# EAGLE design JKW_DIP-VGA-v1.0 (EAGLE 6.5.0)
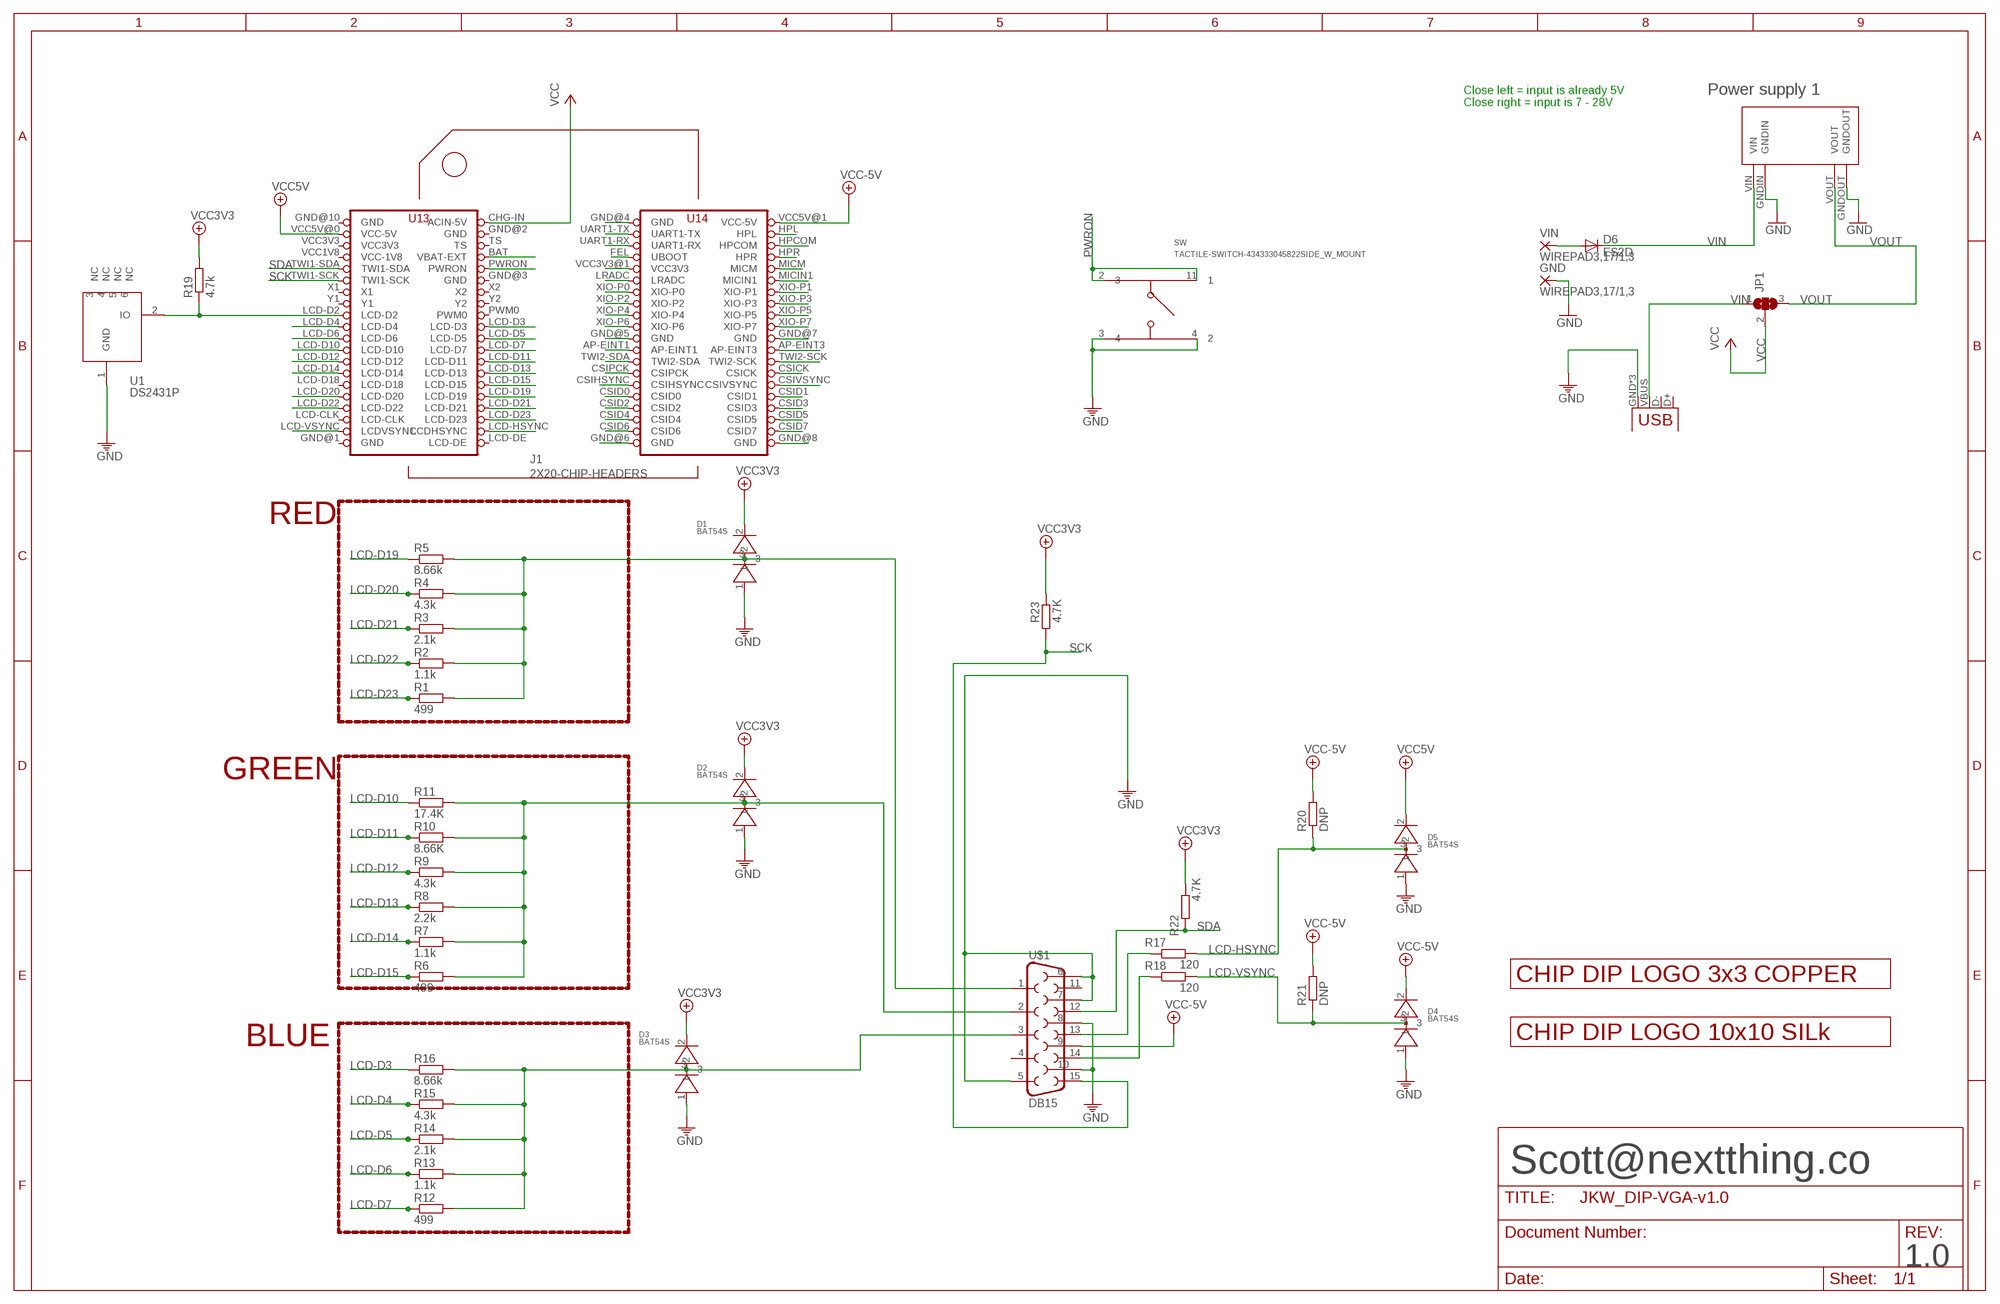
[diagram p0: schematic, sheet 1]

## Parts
D1  BAT54S  [SOT23-BEC]
D2  BAT54S  [SOT23-BEC]
D3  BAT54S  [SOT23-BEC]
D4  BAT54S  [SOT23-BEC]
D5  BAT54S  [SOT23-BEC]
D6  ES2D  [SMB]
GND  WIREPAD3,17/1,3  [3,17/1,3]
J1  2X20-CHIP-HEADERS  [2X20CHIP_SM]
JP1  SJ2W  [SJ_2]
R1  499  R-EU_R0805  [R0805]
R2  1.1k  R-EU_R0805  [R0805]
R3  2.1k  R-EU_R0805  [R0805]
R4  4.3k  R-EU_R0805  [R0805]
R5  8.66k  R-EU_R0805  [R0805]
R6  499  R-EU_R0805  [R0805]
R7  1.1k  R-EU_R0805  [R0805]
R8  2.2k  R-EU_R0805  [R0805]
R9  4.3k  R-EU_R0805  [R0805]
R10  8.66K  R-EU_R0805  [R0805]
R11  17.4K  R-EU_R0805  [R0805]
R12  499  R-EU_R0805  [R0805]
R13  1.1k  R-EU_R0805  [R0805]
R14  2.1k  R-EU_R0805  [R0805]
R15  4.3k  R-EU_R0805  [R0805]
R16  8.66k  R-EU_R0805  [R0805]
R17  120  R-EU_R0805  [R0805]
R18  120  R-EU_R0805  [R0805]
R19  4.7k  R-EU_R0805  [R0805]
R20  DNP  R-EU_R0805  [R0805]
R21  DNP  R-EU_R0805  [R0805]
R22  4.7K  R-EU_R0805  [R0805]
R23  4.7K  R-EU_R0805  [R0805]
SW  TACTILE-SWITCH-434333045822SIDE_W_MOUNT  [TACTILE-SWITCH-K2-1114UA-AW]
U1  DS2431P  [TSOC6]
U$1  DB15  [DB15]
U$5  LOGO_3X3_COPPER  [LOGO_3X3_COPPER]
U$6  LOGO_10X10_SILK  [LOGO_10X10_SILK]
U$9  MP1584EN  [MP1584EN]
USB  USBUSB-MICROB-SMT-DIP  [USB-MICROB-SMT-DIP]
VIN  WIREPAD3,17/1,3  [3,17/1,3]

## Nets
1: J1.CSIVSYNC
AP-EINT1: J1.AP-EINT1
AP-EINT3: J1.AP-EINT3
BAT: J1.BAT(VBAT-EXT)
CSICK: J1.CSICK
CSID0: J1.CSID0
CSID1: J1.CSID1
CSID2: J1.CSID2
CSID3: J1.CSID3
CSID4: J1.CSID4
CSID5: J1.CSID5
CSID6: J1.CSID6
CSID7: J1.CSID7
CSIHSYNC: J1.CSIHSYNC
CSPICK: J1.CSIPCK
FEL: J1.FEL(UBOOT)
GND: D1.1 D2.1 D3.1 D4.1 D5.1 GND.1(P) J1.GND@4(GND) J1.GND@5(GND) J1.GND@6(GND) J1.GND@7(GND) J1.GND@8(GND) SW.3 SW.4 U1.1(GND) U$1.5 U$1.6 U$1.7 U$1.8 U$1.10 U$9.GNDIN U$9.GNDOUT USB.GND USB.MT1(GND) USB.MT2(GND)
HPCOM: J1.HPCOM
HPL: J1.HPL
HPR: J1.HPR
LCD-D3: J1.LCD-D3 R16.1
LCD-D4: J1.LCD-D4 R15.1
LCD-D5: J1.LCD-D5 R14.1
LCD-D6: J1.LCD-D6 R13.1
LCD-D7: J1.LCD-D7 R12.1
LCD-D10: J1.LCD-D10 R11.1
LCD-D11: J1.LCD-D11 R10.1
LCD-D12: J1.LCD-D12 R9.1
LCD-D13: J1.LCD-D13 R8.1
LCD-D14: J1.LCD-D14 R7.1
LCD-D15: J1.LCD-D15 R6.1
LCD-D19: J1.LCD-D19 R5.1
LCD-D20: J1.LCD-D20 R4.1
LCD-D21: J1.LCD-D21 R3.1
LCD-D22: J1.LCD-D22 R2.1
LCD-D23: J1.LCD-D23 R1.1
LCD-HSYNC: D5.3 J1.LCD-HSYNC(LCDHSYNC) R17.2 R20.1
LCD-VSYNC: D4.3 J1.LCD-VSYNC(LCDVSYNC) R18.2 R21.1
LRADC: J1.LRADC
MICIN1: J1.MICIN1
MICM: J1.MICM
N$1: R17.1 U$1.13
N$2: R18.1 U$1.14
N$3: JP1.1 USB.VBUS
N$5: J1.LCD-D2 R19.1 U1.2(IO)
N$12: D2.3 R6.2 R7.2 R8.2 R9.2 R10.2 R11.2 U$1.2
N$13: D1.3 R1.2 R2.2 R3.2 R4.2 R5.2 U$1.1
N$19: D3.3 R12.2 R13.2 R14.2 R15.2 R16.2 U$1.3
N$65: D6.A VIN.1(P)
PWRON: J1.PWRON SW.2 SW.11
SCK: J1.TWI1-SCK R23.1 U$1.15
SDA: J1.TWI1-SDA R22.1 U$1.12
TWI2-SCK: J1.TWI2-SCK
TWI2-SDA: J1.TWI2-SDA
UART1-RX: J1.UART1-RX
UART1-TX: J1.UART1-TX
VCC: J1.CHG-IN(ACIN-5V) JP1.2
VCC3V3: D1.2 D2.2 D3.2 J1.VCC3V3@1(VCC3V3) R19.2 R22.2 R23.2
VCC5V: D4.2 D5.2 J1.VCC5V@0(VCC-5V) J1.VCC5V@1(VCC-5V) R20.2 R21.2 U$1.9 ; supply symbol labelled VCC-5V
VIN: D6.C U$9.VIN
VOUT: JP1.3 U$9.VOUT
XIO-P0: J1.XIO-P0
XIO-P1: J1.XIO-P1
XIO-P2: J1.XIO-P2
XIO-P3: J1.XIO-P3
XIO-P4: J1.XIO-P4
XIO-P5: J1.XIO-P5
XIO-P6: J1.XIO-P6
XIO-P7: J1.XIO-P7
Unconnected: J1.LCD-CLK J1.LCD-D18 J1.LCD-DE J1.PWM0 J1.TS J1.X1 J1.X2 J1.Y1 J1.Y2 U1.3(NC) U1.4(NC) U1.5(NC) U1.6(NC) U$1.4 U$1.11 USB.D+ USB.D-

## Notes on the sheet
- Power supply 1
- Close left = input is already 5V
  Close right = input is 7 - 28V
- RED
- GREEN
- BLUE
- Scott@nextthing.co
- 1.0

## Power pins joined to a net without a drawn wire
GND: J1.GND@1(GND) J1.GND@2(GND) J1.GND@3(GND) J1.GND@10(GND)
VCC3V3: J1.VCC3V3
VCC-1V8: J1.VCC1V8(VCC-1V8)

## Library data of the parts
D1-D5 = VGA-DIP:BAT54S
D6 = diode:ES2D: DIODE
GND VIN = wirepad:WIREPAD: Wire PAD connect wire on PCB
J1 = VGA-DIP:2X20-CHIP-HEADERS: Through hole layout with chip reference
JP1 = jumper:SJ2W: SMD solder JUMPER
R1-R23 = rcl:R-EU_: RESISTOR, European symbol
SW = cheeper:TACTILE-SWITCH-434333045822
U1 = VGA-DIP:DS2431: 1024-Bit EEPROM This chip provides a 4x256 Bit EEPROM, which can be programmed@5V. Write protection and OTP emulation are available, too. Author: Jan Kandziora <jjj@gmx.de>; DESCRIPTION: IC, 1024-Bit, 1-Wire EEPROM, TSOC6; FOOTPRINT: TSOC6; LINK: http://www.digikey.com/product-detail/en/DS2431P%2BT%26R/DS2431P%2BT%26RCT-ND/3647900; MFG: DIGIKEY; MFG_PN: DS2431P+T&RCT-ND; PART_TYPE: IC; PRICE: 0.98; VENDOR: MAXIM; VENDOR_PART_NUMBER: DS2431P+T&R
U$1 = SparkFun-Connectors:DB15: DB15 / VGA right angle through-hole female connector.
U$5 = logo:LOGO_3X3_COPPER
U$6 = logo:LOGO_10X10_SILK
U$9 = power_supply:MP1584EN
USB = Spark:USB

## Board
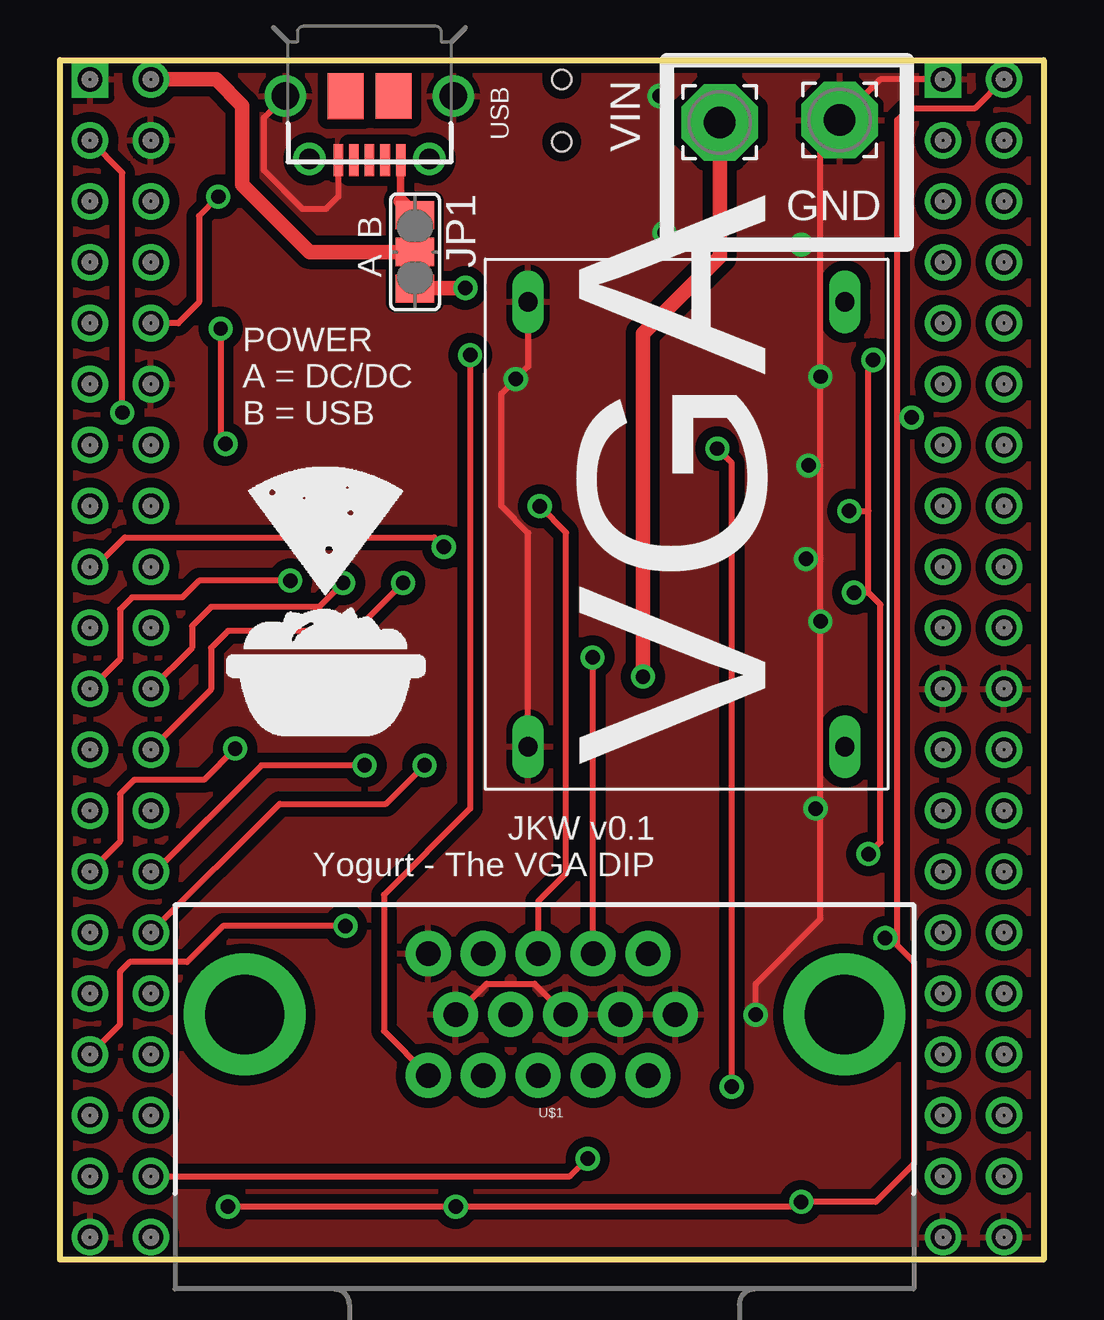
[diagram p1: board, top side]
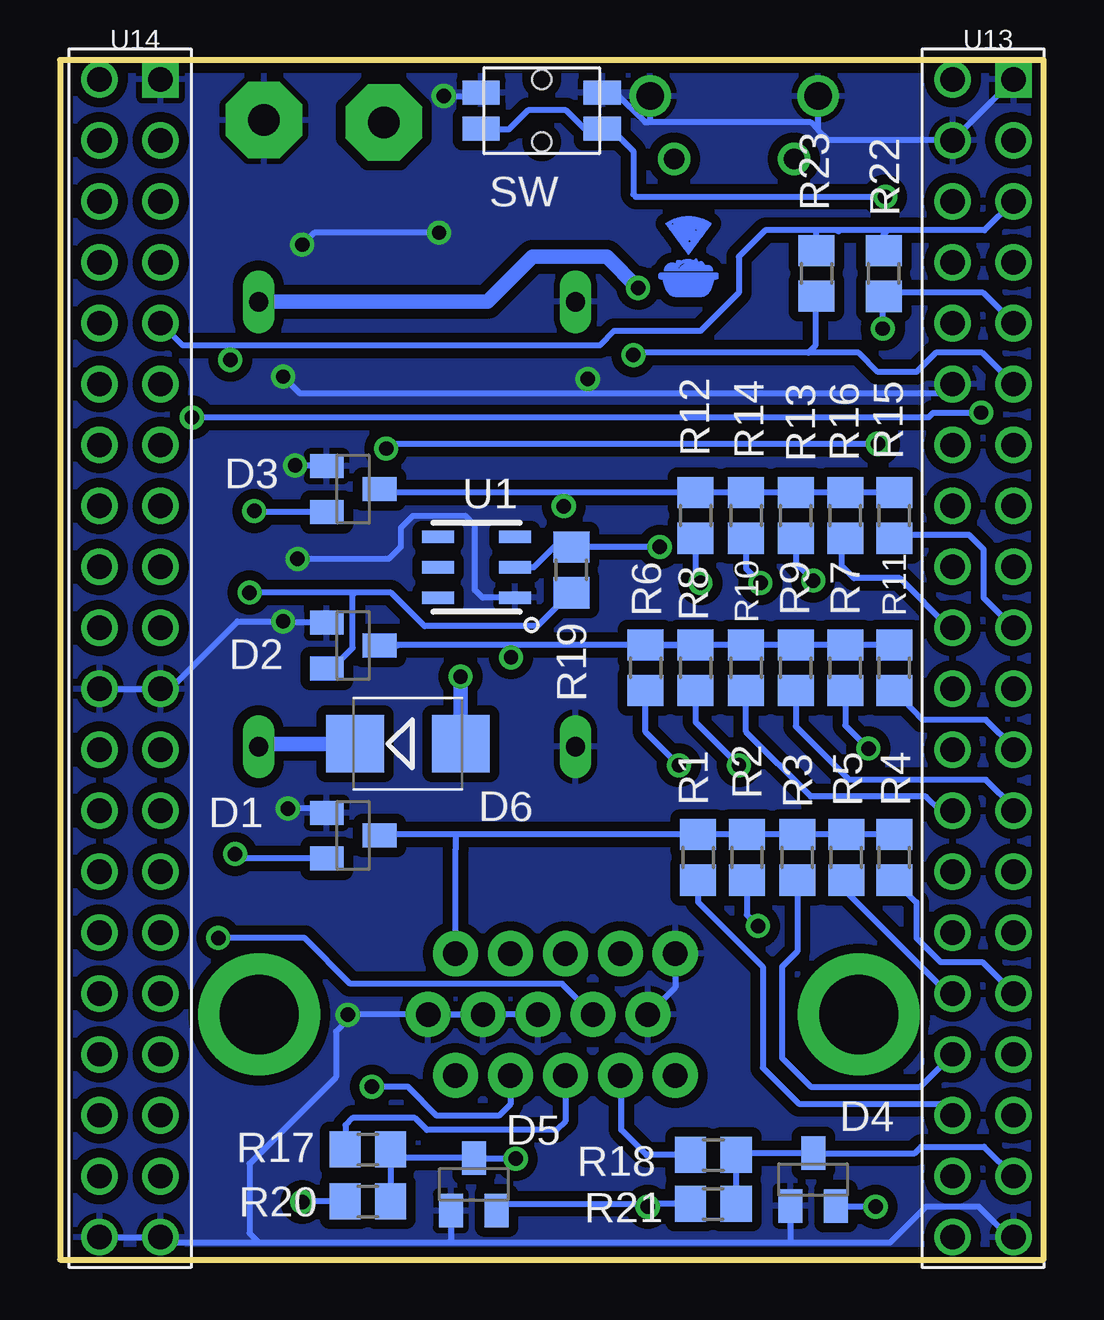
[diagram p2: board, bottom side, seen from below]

Size 41 x 50 mm. Coordinates in mm from the lower left corner, seen from the top.
Outline: 41,0 0,0 0,50 41,50 41,0
Copper layers (1*2*15*16): Top 0.035mm / dielectric 0.2mm / Route2 0.035mm / dielectric 0.2mm / Route15 0.035mm / dielectric 0.2mm / Bottom 0.035mm
Design rules "Hampoo *": minimum track width 3mil, minimum drill 8mil, track to track 3mil, track to pad 3mil, pad to pad 3mil, via to via 3mil, smd to smd 3mil, copper to edge 10mil, drill to drill 8mil, minimum pad ring 10mil, minimum via ring 8mil, stop-mask expansion 4mil, vias tented up to drill 39mil, thermal gap 10mil

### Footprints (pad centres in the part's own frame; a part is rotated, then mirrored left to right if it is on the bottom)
SOT23-BEC = smd 1 x 1.4: 1 -0.95,-1.1; 2 0.95,-1.1; 3 0,1.1
SMB = smd 2.4 x 2.4: A 2.2,0; C -2.2,0
3,17/1,3 = drill 1.321 pad 3.175 octagon: 1 0,0
2X20CHIP_SM = drill 1.016: AP-EINT1 36.81,21.65; AP-EINT3 39.35,21.65; BAT 3.79,41.97; CHG-IN 3.79,49.59; CSICK 39.35,16.57; CSID0 36.81,11.49; CSID1 39.35,11.49; CSID2 36.81,8.95; CSID3 39.35,8.95; CSID4 36.81,6.41; CSID5 39.35,6.41; CSID6 36.81,3.87; CSID7 39.35,3.87; CSIHSYNC 36.81,14.03; CSIPCK 36.81,16.57; CSIVSYNC 39.35,14.03; FEL 36.81,41.97; GND@1 3.79,36.89; GND@2 1.25,1.33; GND@4 39.35,24.19; GND@5 39.35,1.33; GND@6 36.81,1.33; GND@7 36.81,24.19; GND@10 3.79,47.05; HPCOM 39.35,44.51; HPL 39.35,47.05; HPR 39.35,41.97; LCD-CLK 1.25,6.41; LCD-D2 1.25,29.27; LCD-D3 3.79,26.73; LCD-D4 1.25,26.73; LCD-D5 3.79,24.19; LCD-D6 1.25,24.19; LCD-D7 3.79,21.65; LCD-D10 1.25,21.65; LCD-D11 3.79,19.11; LCD-D12 1.25,19.11; LCD-D13 3.79,16.57; LCD-D14 1.25,16.57; LCD-D15 3.79,14.03; LCD-D18 1.25,14.03; LCD-D19 3.79,11.49; LCD-D20 1.25,11.49; LCD-D21 3.79,8.95; LCD-D22 1.25,8.95; LCD-D23 3.79,6.41; LCD-DE 3.79,1.33; LCD-HSYNC 3.79,3.87; LCD-VSYNC 1.25,3.87; LRADC 36.81,36.89; MICIN1 39.35,36.89; MICM 39.35,39.43; PWM0 3.79,29.27; PWRON 3.79,39.43; TS 3.79,44.51; TWI1-SCK 1.25,36.89; TWI1-SDA 1.25,39.43; TWI2-SCK 39.35,19.11; TWI2-SDA 36.81,19.11; UART1-RX 36.81,44.51; UART1-TX 36.81,47.05; VCC1V8 1.25,41.97; VCC3V3 1.25,44.51; VCC3V3@1 36.81,39.43; VCC5V@0 1.25,47.05; VCC5V@1 39.35,49.59; X1 1.25,34.35; X2 3.79,34.35; XIO-P0 36.81,34.35; XIO-P1 39.35,34.35; XIO-P2 36.81,31.81; XIO-P3 39.35,31.81; XIO-P4 36.81,29.27; XIO-P5 39.35,29.27; XIO-P6 36.81,26.73; XIO-P7 39.35,26.73; Y1 1.25,31.81; Y2 3.79,31.81 | drill 1.016 square: GND@3 1.25,49.59; GND@8 36.81,49.59
SJ_2 = smd 1.168 x 1.6: 1 -1.524,0; 2 0,0; 3 1.524,0
R0805 = smd 1.3 x 1.5: 1 -0.95,0; 2 0.95,0
TACTILE-SWITCH-K2-1114UA-AW = smd 1.55 x 1: 2 -2.525,0.75; 3 -2.525,-0.75; 4 2.525,-0.75; 11 2.525,0.75 | hole 0.8: 0,1.3; 0,-1.3
TSOC6 = smd 0.53 x 1.33: 1 -1.27,-1.6; 2 0,-1.6; 3 1.27,-1.6; 4 1.27,1.6; 5 0,1.6; 6 -1.27,1.6
DB15 = drill 1.016 pad 1.88: 1 -4.32,-7.62; 2 -2.03,-7.62; 3 0.26,-7.62; 4 2.55,-7.62; 5 4.84,-7.62; 6 -5.46,-5.08; 7 -3.17,-5.08; 8 -0.88,-5.08; 9 1.41,-5.08; 10 3.7,-5.08; 11 -4.32,-2.54; 12 -2.03,-2.54; 13 0.26,-2.54; 14 2.55,-2.54; 15 4.84,-2.54 | drill 3.302 pad 5.08: G1 -12.5,-5.08; G2 12.5,-5.08
MP1584EN = drill 0.8 long: GNDIN 1.778,14.986; GNDOUT 20.32,14.986; VIN 1.778,1.778; VOUT 20.32,1.778
USB-MICROB-SMT-DIP = smd 0.4 x 1.35: D+ 0,2.675; D- -0.65,2.675; GND 1.3,2.675; ID 0.65,2.675; VBUS -1.3,2.675 | drill 1.15 pad 1.7: MT1 -3.5,0; MT2 3.5,0 | drill 0.85 pad 1.25: MT3 -2.5,2.625; MT4 2.5,2.625 | smd 1.5 x 1.9: P$1 -1,0; P$2 1,0.01

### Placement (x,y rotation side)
D1  28.78,17.68 270 bottom
D2  28.78,25.6 270 bottom
D3  28.78,32.12 270 bottom
D4  9.6,3.33 0 bottom
D5  23.75,3.13 0 bottom
D6  26.5,21.5 0 bottom
GND  32.5,47.5 0 top
J1  0,-0.4 0 top
JP1  14.8,42 270 top
R1  14.4,16.76 90 bottom
R2  12.37,16.76 90 bottom
R3  10.27,16.76 90 bottom
R4  6.22,16.76 90 bottom
R5  8.22,16.76 90 bottom
R6  16.59,24.66 90 bottom
R7  8.27,24.66 90 bottom
R8  14.51,24.66 90 bottom
R9  10.32,24.66 90 bottom
R10  12.4,24.66 90 bottom
R11  6.22,24.66 90 bottom
R12  14.51,31.01 90 bottom
R13  10.32,31.01 90 bottom
R14  12.4,31.01 90 bottom
R15  6.22,31.01 90 bottom
R16  8.27,31.01 90 bottom
R17  28.16,4.59 0 bottom
R18  13.76,4.35 0 bottom
R19  19.69,28.75 270 bottom
R20  28.17,2.42 180 bottom
R21  13.77,2.32 180 bottom
R22  6.67,41.1 90 bottom
R23  9.47,41.1 90 bottom
SW  20.92,47.89 180 bottom
U1  23.63,28.86 90 bottom
U$1  20.19,5.13 180 top
U$5  14.8,41.8 0 bottom
U$6  6.9,21.8 0 top
U$9  34.5,19.6 90 top
USB  12.9,48.5 180 top
VIN  27.5,47.4 0 top

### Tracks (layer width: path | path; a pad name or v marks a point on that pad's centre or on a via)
GND  (via drill 0.6)
  Top 0.254: U$1.10 17.78,11.5 19.78,11.5 U$1.8 | 31.7,29.2 v31.7,26.6 31.7,19 | 31.7,29.2 31.7,33.1 | 31.7,33.1 v31.7,36.8 31.7,42.3 | v31.2,33.1 31.7,33.1 | v31.5,18.8 31.7,19 | v29,10.2 29,11.5 31.7,14.2 31.7,19 | v31.1,29.2 31.7,29.2 | USB.GND 11.6,44.3 11.1,43.8 10.1,43.8 8.5,45.4 8.5,47.6 USB.MT2 | v30.9,42.3 31.7,42.3 | U$9.GNDIN 19.51,30.29 18.4,31.4 18.4,36.1 v19,36.7 19.51,37.21 U$9.GNDOUT | 31.7,42.3 31.7,46.7 GND.1 34.19,49.19 J1.GND@8 | v25.2,42.8 25.2,48.3 v25,48.5
  Bottom 0.254: U$1.8 U$1.7 U$1.6 28.79,10.21 28.8,10.2 | J1.GND@5 J1.GND@6 36.58,0.7 32.7,0.7 | J1.GND@2 1.43,0.93 2.7,2.2 4.9,2.2 6.4,0.7 10.6,0.7 | 10.6,0.7 24.8,0.7 | 24.8,0.7 32.7,0.7 | D4.1 10.55,0.75 10.6,0.7 | D5.1 24.7,0.8 24.8,0.7 | 28.8,10.2 29.5,9.5 29.5,7.6 33.1,4 33.1,1.1 32.7,0.7 | U$1.5 15.35,11.35 U$1.10 | D2.1 31.64,26.55 v31.7,26.6 33.6,26.6 36.41,23.79 J1.GND@7 J1.GND@4 | D3.1 29.91,33.1 v31.2,33.1 | D1.1 30.05,18.8 v31.5,18.8 | 28.8,10.2 v29,10.2 | J1.GND@3 J1.GND@10 8.95,46.65 9.4,47.1 | J1.GND@1 4.18,36.1 19,36.1 | 19,36.1 31,36.1 v31.7,36.8 | U1.1 23.39,27.59 23.7,27.9 23.7,30.6 24.1,31 26.3,31 26.8,30.5 26.8,29.7 27.3,29.2 v31.1,29.2 | 9.4,47.1 9.7,47.4 16.5,47.4 | USB.MT2 9.4,47.1 | USB.MT1 16.4,47.5 16.5,47.4 | 16.5,47.4 16.6,47.4 17.84,48.64 SW.3 | v19,36.7 19,36.1 | v25,48.5 23.58,48.5 SW.4 | v25.2,42.8 30.4,42.8 v30.9,42.3
  pour Top (isolate 0.406): 0,0 41,0 41,50 0,50
  pour Bottom (isolate 0.406): 0,0 41,0 41,50 0,50
LCD-D3
  Bottom 0.254: J1.LCD-D3 3.93,26.33 6,28.4 7.9,28.4 8.4,28.9 8.4,30.04 R16.1
LCD-D4
  Bottom 0.254: J1.LCD-D4 2.5,27.58 2.5,29.6 3.1,30.2 6.25,30.2 R15.1
LCD-D5  (via drill 0.6)
  Top 0.254: v11.8,28.2 10.8,27.2 6.3,27.2 5.5,26.4 5.5,25.5 J1.LCD-D5
  Bottom 0.254: R14.1 12.4,28.8 v11.8,28.2
LCD-D6  (via drill 0.6)
  Top 0.254: v9.6,28.3 5.8,28.3 5.1,27.6 3,27.6 2.5,27.1 2.5,25.04 J1.LCD-D6
  Bottom 0.254: R13.1 10.32,29.03 v9.6,28.3
LCD-D7  (via drill 0.6)
  Top 0.254: v14.3,28.2 12.3,26.2 7,26.2 6.3,25.5 6.3,23.76 J1.LCD-D7
  Bottom 0.254: R12.1 14.51,28.41 v14.3,28.2
LCD-D10
  Bottom 0.254: J1.LCD-D10 1.25,21.35 2.4,22.5 5.05,22.5 R11.1
LCD-D11
  Bottom 0.254: J1.LCD-D11 4.31,18.71 4.9,19.3 9.7,19.3 12.4,22 R10.1
LCD-D12
  Bottom 0.254: J1.LCD-D12 1.25,18.85 2.4,20 8.1,20 10.1,22 10.2,22.1 10.32,22.23 R9.1
LCD-D13  (via drill 0.6)
  Top 0.254: v12.7,20.6 8.4,20.6 3.97,16.17 J1.LCD-D13
  Bottom 0.254: R8.1 14.51,22.41 v12.7,20.6
LCD-D14  (via drill 0.6)
  Top 0.254: v7.3,21.3 6,20 3.1,20 2.5,19.4 2.5,17.42 J1.LCD-D14
  Bottom 0.254: R7.1 8.27,22.27 v7.3,21.3
LCD-D15  (via drill 0.6)
  Top 0.254: J1.LCD-D15 9.16,19 13.6,19 v15.2,20.6
  Bottom 0.254: v15.2,20.6 16.59,21.99 R6.1
LCD-D19
  Bottom 0.254: J1.LCD-D19 3.99,11.09 8.22,15.32 R5.1
LCD-D20
  Bottom 0.254: R4.1 5.3,14.89 5.3,13.4 4.3,12.4 2.56,12.4 J1.LCD-D20
LCD-D21
  Bottom 0.254: R3.1 10.27,12.83 10.9,12.2 10.9,8.4 9.7,7.2 5.14,7.2 J1.LCD-D21
LCD-D22  (via drill 0.6)
  Top 0.254: v11.9,13.9 6.8,13.9 5.3,12.4 2.9,12.4 2.65,12.15 2.6,12.1 2.5,12 2.5,9.8 J1.LCD-D22
  Bottom 0.254: R2.1 12.37,14.37 v11.9,13.9
LCD-D23
  Bottom 0.254: R1.1 14.4,14.9 11.7,12.2 11.7,8 10.2,6.5 4.28,6.5 J1.LCD-D23
LCD-HSYNC  (via drill 0.6)
  Top 0.254: J1.LCD-HSYNC 21.27,3.47 v22,4.2
  Bottom 0.254: R20.1 R17.2 26.86,4.23 D5.3 23.71,4.2 v22,4.2
LCD-VSYNC
  Bottom 0.254: J1.LCD-VSYNC 2.48,4.7 5.1,4.7 5.37,4.43 D4.3 12.73,4.43 R18.2 R21.1
N$1
  Bottom 0.254: U$1.13 19.93,5.77 20.3,5.4 25.7,5.4 26.2,5.9 28.8,5.9 29.1,5.6 29.1,4.6 R17.1
N$2
  Bottom 0.254: R18.1 16.55,4.35 17.6,5.4 17.6,7.63 U$1.14
N$3
  Top 0.305: USB.VBUS 14.2,44.12
  Top 0.61: 14.2,44.12 JP1.1
N$5  (via drill 0.6)
  Top 0.254: J1.LCD-D2 1.47,28.87 2.7,30.1 15.6,30.1 v16,29.7
  Bottom 0.254: U1.2 21.25,28.86 20.4,29.7 R19.1 v16,29.7
N$12  (via drill 0.6)
  Top 0.254: v22.2,25.1 22.22,25.08 U$1.2
  Bottom 0.254: R11.2 R7.2 R9.2 R10.2 R6.2 R8.2 22.2,25.61 | 22.2,25.61 26.9,25.61 | 26.9,25.61 26.99,25.61 27,25.6 | D2.3 26.92,25.6 26.9,25.61 | v22.2,25.1 22.2,25.61
N$13
  Bottom 0.254: R4.2 R5.2 R3.2 R2.2 R1.2 24.5,17.71 | 24.5,17.71 27.59,17.71 27.62,17.68 D1.3 | 24.5,17.71 24.5,17.1 24.51,17.09 U$1.1
N$19  (via drill 0.6)
  Top 0.254: 19.93,31.33 v20,31.4 21.1,30.3 21.1,16.1 19.93,14.93 U$1.3
  Bottom 0.254: R16.2 R13.2 R14.2 R12.2 20,31.96 | 20,31.96 27.53,31.96 D3.3 | R15.2 R16.2 | R16.2 8.27,31.94 8.3,31.9 | v20,31.4 20,31.96
N$65  (via drill 0.6)
  Top 0.61: v24.3,24.3 24.3,38.6 27.5,41.8 VIN.1
  Bottom 0.61: D6.A v24.3,24.3
PWRON  (via drill 0.6)
  Top 0.254: v6.6,44.3 5.8,43.5 5.8,39.9 4.93,39.03 J1.PWRON
  Bottom 0.254: v6.6,44.3 17,44.3 17.1,44.4 17.1,46.2 18.04,47.14 SW.2 19.14,47.14 19.9,47.9 21.5,47.9 22.3,47.1 23.41,47.1 SW.11
SCK  (via drill 0.6)
  Top 0.254: v17.1,37.7 17.1,18.8 13.5,15.2 13.5,9.52 U$1.15
  Bottom 0.254: J1.TWI1-SCK 2.56,37.8 4.5,37.8 5.3,37 6.9,37 7.7,37.8 9.8,37.8 | 9.5,40.12 R23.1 9.52,40.2 9.52,38.09 9.8,37.8 | 9.8,37.8 17,37.8 v17.1,37.7
SDA  (via drill 0.6)
  Top 0.254: v28,7.2 28,33.2 v27.4,33.8 | v6.7,38.8 6.7,34.2 arc90 v6.9,34
  Bottom 0.254: J1.TWI1-SDA 2.52,40.3 6.61,40.3 R22.1 6.7,40.11 v6.7,38.8 | U$1.12 22.22,6.48 22.7,6 25.3,6 26.5,7.2 v28,7.2 | v6.9,34 27.2,34 arc-90 v27.4,33.8
VCC
  Top 0.61: J1.CHG-IN 6.51,49.19 7.6,48.1 7.6,44.8 10.4,42 JP1.2
VCC3V3  (via drill 0.6)
  Top 0.254: 33.7,27.8 33.7,31.2 | v32.9,31.2 33.7,31.2 | v33.1,27.8 33.7,27.8 | 33.7,27.8 34.2,27.3 34.2,17.4 v33.7,16.9 | 33.7,31.2 33.7,37.3 v33.9,37.5
  Bottom 0.254: J1.VCC3V3 2.46,42.9 6.5,42.9 | 6.5,42.9 8.6,42.9 | 8.6,42.9 9.5,42.9 | 8.55,42.85 8.6,42.9 | R22.2 6.67,42.73 6.5,42.9 | R23.2 9.47,42.87 9.5,42.9 | D1.2 33.52,16.73 v33.7,16.9 | 36.74,39.1 J1.VCC3V3@1 35.88,38.1 33.9,38.1 | D3.2 32.87,31.17 v32.9,31.2 | 9.5,42.9 11.6,42.9 12.7,41.8 12.7,40.3 14.3,38.7 17.9,38.7 18.5,38.1 33.9,38.1 | R19.2 19.7,27.8 21.1,26.4 25.8,26.4 27.2,27.8 28.7,27.8 | 28.7,27.8 v33.1,27.8 | D2.2 29.66,24.65 28.8,25.5 28.8,27.7 28.7,27.8 | v33.9,37.5 33.9,38.1
VCC5V  (via drill 0.6)
  Top 0.254: 34.9,13.4 34.9,13.1 35.6,12.4 35.6,4 34,2.4 v30.9,2.4 30.7,2.2 v16.5,2.2 v7,2.2 | 34.9,13.4 34.9,35.1 | 34.9,35.1 34.9,47.5 35.4,48 38.16,48 J1.VCC5V@1 | v34.4,13.4 34.9,13.4 | v35.5,35.1 34.9,35.1 | v2.6,35.3 2.6,45.3 J1.VCC5V@0
  Bottom 0.254: U$1.9 20.07,11.5 28.9,11.5 30.8,13.4 v34.4,13.4 | R20.2 30.88,2.42 v30.9,2.4 | v35.5,35.1 4.8,35.1 4.6,35.3 v2.6,35.3 | D5.2 22.87,2.03 | 22.87,2.03 22.9,2 | v7,2.2 8.62,2.2 D4.2 | R21.2 16.38,2.32 | 16.38,2.32 v16.5,2.2 | 22.87,2.03 22.58,2.32 16.38,2.32
VIN
  Bottom 0.61: D6.C 32.6,21.5 arc-90 U$9.VIN
VOUT  (via drill 0.6)
  Top 0.61: v16.9,40.5 14.82,40.5 JP1.3
  Bottom 0.61: U$9.VOUT 23.18,39.92 21.3,41.8 18.2,41.8 v16.9,40.5

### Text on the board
tNames: B | A | POWER / A = DC/DC / B = USB | VGA | JKW v0.1 / Yogurt - The VGA DIP

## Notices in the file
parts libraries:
SparkFun-Connectors: Licensing: Creative Commons ShareAlike 4.0 International - https://creativecommons.org/licenses/by-sa/4.0
